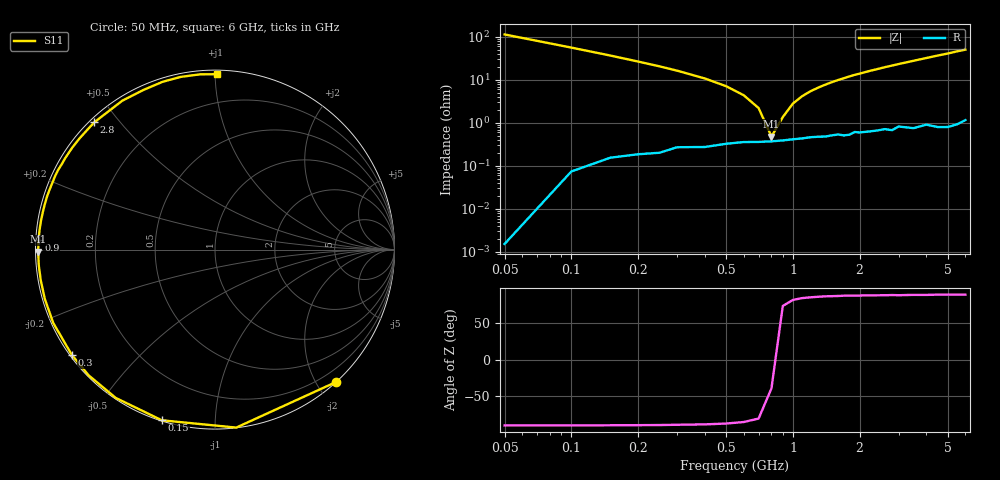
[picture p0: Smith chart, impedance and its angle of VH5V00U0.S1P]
! Infineon Technologies  Discrete & RF Semiconductors
! BB 814
! Si Tuning Diode in SOT23
! VR = 5 V
! S-Parameters:  July  1999
# GHz  S  MA  R  50
!  f  S11
! GHz  MAG  ANG
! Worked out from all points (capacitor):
!   34 points, 50 MHz to 6 GHz, reference 50 ohm
!   read as one part to ground: C = 27.9 pF near 50 MHz
!   lowest |Z| = 482 mohm at 800 MHz (marker M1)
!   series resonance near 818.9 MHz, so ESL is about 1.4 nH
!   S11 on the Smith chart (normalised r, x): 50 MHz: 0.00, -2.27; 150 MHz: 0.00, -0.74; 300 MHz: 0.01, -0.33; 900 MHz: 0.01, +0.03; 2.8 GHz: 0.01, +0.43; 6 GHz: 0.02, +1.01
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0.05  1 -47.5
0.1  0.9987 -83.2
0.15  0.996 -107.3
0.2  0.9942 -123.8
0.25  0.9931 -135.1
0.3  0.9902 -143.7
0.4  0.9895 -155.6
0.5  0.9872 -163.8
0.6  0.9858 -170.0
0.7  0.9857 -175.0
0.8  0.9852 -179.3
0.9  0.9845 177.0
1  0.9835 173.6
1.2  0.9818 167.6
1.4  0.9814 162.4
1.6  0.9795 157.5
1.7  0.9806 155.3
1.9  0.9772 150.7
2.2  0.9773 144.6
2.4  0.9767 140.8
2.8  0.9774 133.5
3  0.9732 129.9
3.5  0.9772 121.9
4  0.9746 114.3
4.5  0.9794 107.3
5  0.981 101.2
5.5  0.9801 94.8
6  0.9772 89.5
